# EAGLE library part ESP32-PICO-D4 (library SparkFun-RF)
Espressif ESP32 Pico D4 WiFi-compatible SoC microcontroller. Bluetooth Low energy support (BLE, BT4.0, Bluetooth Smart) 28 GPIO pins Dual-core Tensilica LX6 microprocessor Integrated 4MB SPI flash memory Hardware accelerated encryption (AES, SHA2, ECC, RSA-4096) 520kB internal SRAM
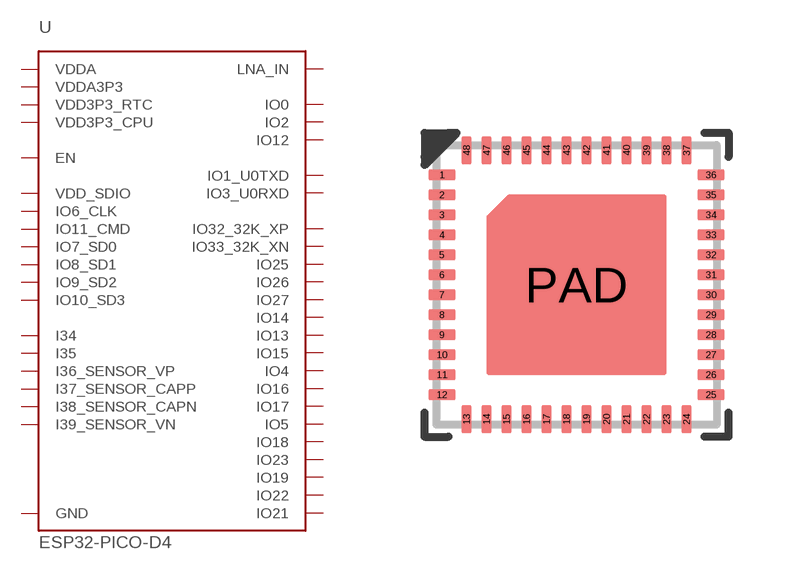
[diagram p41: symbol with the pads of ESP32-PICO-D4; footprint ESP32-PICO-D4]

Designator prefix U

## ESP32-PICO-D4  [ESP32-PICO-D4]
1  VDDA
2  LNA_IN
3  VDDA3P3
4  VDDA3P3
5  I36_SENSOR_VP
6  I37_SENSOR_CAPP
7  I38_SENSOR_CAPN
8  I39_SENSOR_VN
9  EN
10  I34
11  I35
12  IO32_32K_XP
13  IO33_32K_XN
14  IO25
15  IO26
16  IO27
17  IO14
18  IO12
19  VDD3P3_RTC
20  IO13
21  IO15
22  IO2
23  IO0
24  IO4
25  IO16
26  VDD_SDIO
27  IO17
28  IO9_SD2
29  IO10_SD3
30  IO11_CMD
31  IO6_CLK
32  IO7_SD0
33  IO8_SD1
34  IO5
35  IO18
36  IO23
37  VDD3P3_CPU
38  IO19
39  IO22
40  IO3_U0RXD
41  IO1_U0TXD
42  IO21
43  VDDA
46  VDDA
PAD  GND

## Footprint ESP32-PICO-D4 (pad centres in mm)
smd 0.68 x 0.25: 1 -3.365,2.75; 2 -3.365,2.25; 3 -3.365,1.75; 4 -3.365,1.25; 5 -3.365,0.75; 6 -3.365,0.25; 7 -3.365,-0.25; 8 -3.365,-0.75; 9 -3.365,-1.25; 10 -3.365,-1.75; 11 -3.365,-2.25; 12 -3.365,-2.75; 25 3.365,-2.75; 26 3.365,-2.25; 27 3.365,-1.75; 28 3.365,-1.25; 29 3.365,-0.75; 30 3.365,-0.25; 31 3.365,0.25; 32 3.365,0.75; 33 3.365,1.25; 34 3.365,1.75; 35 3.365,2.25; 36 3.365,2.75
smd 0.25 x 0.68: 13 -2.75,-3.365; 14 -2.25,-3.365; 15 -1.75,-3.365; 16 -1.25,-3.365; 17 -0.75,-3.365; 18 -0.25,-3.365; 19 0.25,-3.365; 20 0.75,-3.365; 21 1.25,-3.365; 22 1.75,-3.365; 23 2.25,-3.365; 24 2.75,-3.365; 37 2.75,3.365; 38 2.25,3.365; 39 1.75,3.365; 40 1.25,3.365; 41 0.75,3.365; 42 0.25,3.365; 43 -0.25,3.365; 44 -0.75,3.365; 45 -1.25,3.365; 46 -1.75,3.365; 47 -2.25,3.365; 48 -2.75,3.365
smd 2 x 2: PAD 0,0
